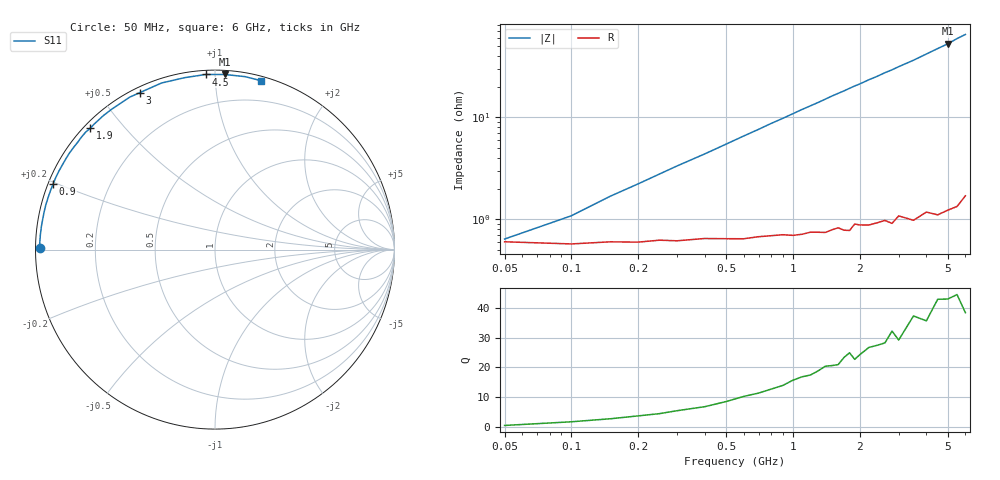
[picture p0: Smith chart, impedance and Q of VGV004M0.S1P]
! Infineon Technologies  Discrete & RF Semiconductors
! BB 831
! Si Tuning Diode in SOD323
! VR =
! S-Parameters:  July  1999
# GHz  S  MA  R  50
!  f  S11
! GHz  MAG  ANG
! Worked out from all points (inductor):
!   34 points, 50 MHz to 6 GHz, reference 50 ohm
!   read as one part to ground: L = 1.72 nH near 200 MHz
!   highest Q = 43.1 at 5 GHz (marker M1), where L = 1.68 nH
!   S11 on the Smith chart (normalised r, x): 50 MHz: 0.01, +0.00; 900 MHz: 0.01, +0.20; 1.9 GHz: 0.02, +0.41; 3 GHz: 0.02, +0.63; 4.5 GHz: 0.02, +0.95; 6 GHz: 0.03, +1.31
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0.05  0.9763 179.5
0.1  0.9774 177.9
0.15  0.9764 176.4
0.3  0.9759 172.5
0.5  0.9749 167.6
0.6  0.9751 165.1
0.8  0.9736 160.2
0.9  0.9733 157.9
1.1  0.9735 153.1
1.3  0.9728 148.7
1.4  0.9732 146.4
1.5  0.9719 144.1
1.6  0.971 142.0
1.7  0.9728 140.0
1.8  0.9734 137.8
1.9  0.9697 135.7
2  0.9707 133.9
2.2  0.9717 129.8
2.4  0.9711 126.3
2.6  0.9706 122.4
2.8  0.9733 119.2
3  0.9696 115.6
3.5  0.9748 107.8
4  0.9728 100.0
4.5  0.977 93.0
5  0.9771 86.8
5.5  0.9782 80.1
6  0.9752 74.9
